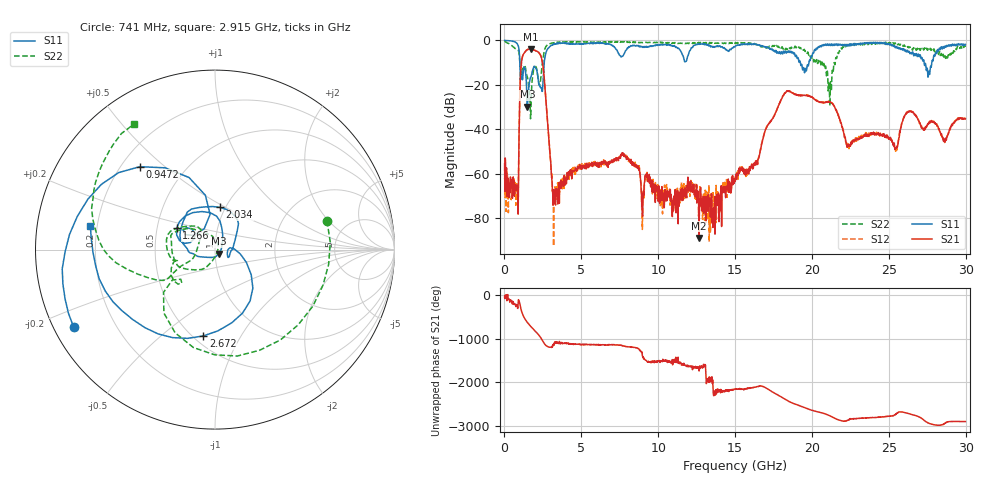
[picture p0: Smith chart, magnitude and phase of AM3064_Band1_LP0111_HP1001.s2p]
# Hz S DB R 50.0
!freq dBS11 angS11 dBS21 angS21 dBS12 angS12 dBS22 angS22
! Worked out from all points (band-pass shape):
!   1600 points, 10 MHz to 29.98 GHz, reference 50 ohm
!   highest |S21| = -3.87 dB at 1.716 GHz (marker M1); lowest = -89.0 dB at 12.66 GHz (marker M2)
!   |S21| within 3 dB of the highest: 1.191 GHz to 2.358 GHz (1.167 GHz wide, 65.8 % of centre)
!   lowest |S11| = -29.9 dB at 1.491 GHz (marker M3), VSWR 1.07, Z = 52.2 - j2.45 ohm
!   |S11| at or under -10 dB: 1.002 GHz to 2.585 GHz (1.583 GHz wide, 88.3 % of centre); 19.24 GHz to 19.8 GHz (554.7 MHz wide, 2.84 % of centre); 27.3 GHz to 27.8 GHz (495.7 MHz wide, 1.8 % of centre)
!   |S22| runs from -35.3 to -0.3 dB; largest |S21 - S12| = 0.0087
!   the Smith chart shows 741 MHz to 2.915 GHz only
!   S11 on the Smith chart (normalised r, x): 741 MHz: 0.06, -0.26; 947.2 MHz: 0.27, +0.42; 1.266 GHz: 0.63, +0.16; 2.034 GHz: 0.94, +0.47; 2.672 GHz: 0.56, -0.70; 2.915 GHz: 0.17, +0.09
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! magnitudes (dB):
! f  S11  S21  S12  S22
! 10 MHz  0.0  -55.6  -62.6  -0.3
! 741 MHz  -0.9  -67.6  -74.2  -3.8
! 947.2 MHz  -4.1  -43.4  -43.3  -5.8
! 1.266 GHz  -12.2  -5.9  -5.8  -11.5
! 1.491 GHz  -29.9  -4.2  -4.1  -16.5
! 1.716 GHz  -16.4  -3.9  -3.9  -33.5
! 2.034 GHz  -12.5  -4.7  -4.6  -11.8
! 2.672 GHz  -6.3  -24.4  -24.5  -3.1
! 2.915 GHz  -3.0  -46.8  -46.5  -1.6
! 3.271 GHz  -1.6  -72.3  -72.6  -1.0
! 5.015 GHz  -1.4  -56.3  -57.1  -0.6
! 7.751 GHz  -6.4  -51.4  -51.5  -0.7
! 10 GHz  -2.1  -72.5  -69.6  -0.9
! 12.66 GHz  -1.6  -89.0  -83.0  -1.1
! 15 GHz  -2.7  -62.3  -62.0  -1.4
! 18.27 GHz  -4.8  -23.6  -23.5  -4.2
! 19.99 GHz  -7.3  -25.5  -25.6  -8.0
! 21.17 GHz  -1.9  -27.6  -27.6  -29.4
! 22.37 GHz  -2.3  -46.8  -46.5  -1.9
! 25 GHz  -1.4  -44.4  -44.5  -1.2
! 27.58 GHz  -14.7  -37.2  -37.4  -3.5
! 29.98 GHz  -1.8  -35.3  -35.1  -2.9
